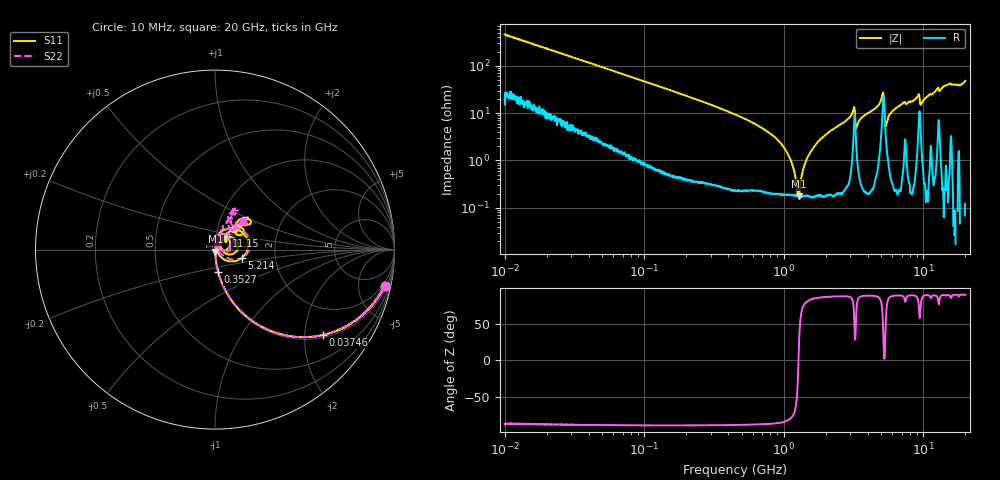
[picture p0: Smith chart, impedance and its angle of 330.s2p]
!Keysight Technologies,P5008B,MY61100088,A.16.20.02
!Date: Friday, August 30, 2024 14:00:04
!Correction: S11(C  2-Port  )
!S21(C  2-Port  )
!S12(C  2-Port  )
!S22(C  2-Port  )
!S2P File: Measurements: S11, S21, S12, S22:Log Frequency Sweep
# Hz S  MA  R 50
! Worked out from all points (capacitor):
!   1601 points, 10 MHz to 20 GHz, reference 50 ohm
!   read as one part in series: C = 34.8 pF near 10.39 MHz
!   lowest |Z| = 176 mohm at 1.278 GHz (marker M1)
!   series resonance near 1.274 GHz, so ESL is about 450 pH
!   S11 on the Smith chart (normalised r, x): 10 MHz: 1.40, -9.14; 37.46 MHz: 1.07, -2.48; 352.7 MHz: 1.00, -0.26; 5.214 GHz: 1.34, -0.13; 11.15 GHz: 1.12, +0.17; 20 GHz: 1.30, +0.42
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1e7  0.968 -12.2  0.2113 75.1  0.2112 75.1  0.9675 -12.2
3.555162e7  0.7833 -36.8  0.5987 51.5  0.5984 51.5  0.7831 -36.8
3.745881e7  0.7687 -38.3  0.6193 50.2  0.619 50.2  0.7687 -38.3
1.263918e8  0.3475 -68.9  0.9322 20.2  0.9317 20.2  0.3476 -68.9
3.526613e8  0.1272 -81.8  0.9892 6.9  0.9889 6.9  0.1272 -81.9
4.472136e8  0.09768 -83.4  0.993 5.1  0.9925 5.1  0.09761 -83.8
8.990775e8  0.03627 -85.1  0.9975 1.1  0.9969 1.1  0.03607 -87.2
1.27782e9  0.01119 -77.7  0.9982 -0.6  0.9979 -0.7  0.01112 -87.1
1.508967e9  0.002987 -16.4  0.9985 -1.5  0.998 -1.5  0.001016 -53.6
1.589917e9  0.003127 41.2  0.9985 -1.8  0.998 -1.8  0.002093 60.5
1.731853e9  0.007689 74.5  0.9986 -2.2  0.998 -2.3  0.007787 73.9
2.09429e9  0.01968 80.8  0.9984 -3.4  0.998 -3.4  0.01933 80.3
3.121338e9  0.07257 72.5  0.9825 -7.9  0.9822 -7.9  0.07378 66.6
3.399988e9  0.02399 79.8  0.9936 -5.6  0.9931 -5.6  0.02547 55.5
5.213871e9  0.1572 -18.1  0.8389 -5.9  0.8385 -6.0  0.173 -11.8
5.652411e9  0.0143 60.1  0.9942 -9.1  0.9937 -9.1  0.0208 45.2
7.133913e9  0.07727 49.1  0.9952 -14.6  0.9947 -14.7  0.07445 89.8
9.132954e9  0.1009 44.2  0.9744 -20.9  0.974 -21.0  0.09614 61.8
9.901129e9  0.03975 44.2  0.9957 -18.7  0.9953 -18.8  0.03581 64.2
1.11497e10  0.09834 50.8  0.9912 -23.4  0.9905 -23.6  0.09579 68.2
1.447892e10  0.2321 46.6  0.9759 -31.1  0.9753 -31.3  0.2301 64.3
2e10  0.2197 43.8  0.9798 -45.1  0.9796 -45.4  0.2258 45.5
